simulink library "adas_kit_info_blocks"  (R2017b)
settings: Solver=ode1  StartTime=0.0  StopTime=Inf  FixedStep=0.001  RelTol=1e-3  EnableMultiTasking=on
PostLoadFcn:
  | , if any(exist('dsrtsu_mdlpostloadfcn', 'file') == [2, 3, 6]), try dsrtsu_mdlpostloadfcn('Execute', bdroot); catch fprintf('Error in PostLoadFcn (dsrtsu_mdlpostloadfcn) for model "%s":\n %s\n', bdroot, lasterr); end, end,
libraries: simulink x10, rtican x2

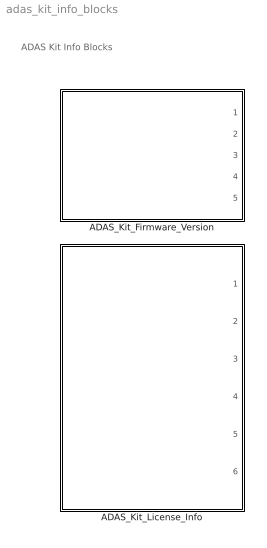
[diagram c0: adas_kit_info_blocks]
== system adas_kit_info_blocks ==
  note: ADAS Kit Info Blocks
  ADAS_Kit_Firmware_Version : Subsystem
  ADAS_Kit_License_Info : Subsystem

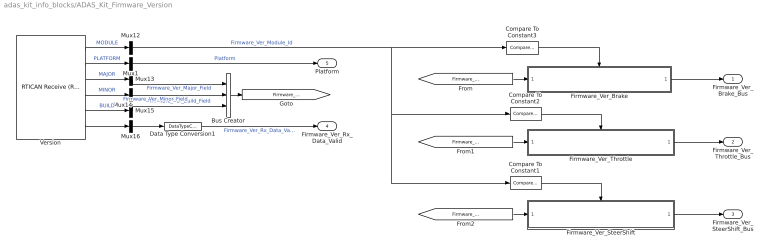
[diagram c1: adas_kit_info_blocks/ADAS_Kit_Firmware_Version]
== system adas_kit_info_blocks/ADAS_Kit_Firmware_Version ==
  Bus Creator : BusCreator  Inputs=3
  Compare To Constant1 : simulink/Logic and Bit Operations/Compare To Constant  relop===  const=3.0  OutDataTypeStr=boolean
  Compare To Constant2 : simulink/Logic and Bit Operations/Compare To Constant  relop===  const=2  OutDataTypeStr=boolean
  Compare To Constant3 : simulink/Logic and Bit Operations/Compare To Constant  relop===  const=1  OutDataTypeStr=boolean
  Data Type Conversion1 : DataTypeConversion  OutDataTypeStr=boolean
  Firmware_Ver_Brake : Subsystem  TreatAsAtomicUnit=on
  Firmware_Ver_SteerShift : Subsystem  TreatAsAtomicUnit=on
  Firmware_Ver_Throttle : Subsystem  TreatAsAtomicUnit=on
  Mux{1,12..16} (6 alike) : Mux  Inputs=1
  Version : rtican/RTICAN Receive (RX)   Reserved1=[]  Reserved2=[]  Reserved3=[]  Reserved4=[]  SfcnMessage=[]  Msg_Struct=[]  BoardTypeNo=[]  BoardNo=[]  ChannelNo=[]  Parameters=[]  DialogFcn=[]  UnitName=[]  Revision=[]  UnitValues=[]  DSProperties=struct('RTI',struct('Version',uint32(5),'BlockType',struct('isSLSource',uint8(1),'isSLSink',uint8(1),'isHWSource',uint8(0),'isHWSink',uint8(0),'isSetup',uint8(0),'isInline',uint8(1),'isNonInline',uint8(0),'isInterrupt',uint8(0),'isChannelwise',uint8(0)),'IOBoardType','RTICAN','UnitType','MESSAGE','Identifier','RX','DialogType','MSVC','BlockSet','RTICAN','SlaveProcessor','CAN'))  RTIBlockInterface=struct('OutputPortsWidth',int32([1 1 1 1 1 1]),'OutputPortsActive',[1 1 1 1 1 1],'OutputPortsName',{{'MODULE','PLATFORM','MAJOR','MINOR','BUILD',['RX status']}},'OutputPortsDataType',{{'SS_UINT8','SS_UINT8','SS_UINT16','SS_UINT16','SS_UINT16','SS_DOUBLE'}},'OutputPortsLabel',{{'MODULE','PLATFORM','MAJOR','MINOR','BUILD',''}},'OutputPortsLabelMode','ON','InputPortsWidth',int32(0),'InputPortsActive'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  RTIBlockParameters=struct('BoardTypeNo',{{1,'OFF',[]}},'BoardNo',{{1,'ON',[1 16]}},'ChannelNo',{{1,'ON',[1 2]}},'Parameters',{{struct('DataFileSupport',struct('DataFileSelectedMaster',1,'DataFileSelectedLocal',1,'DataFileName','c:\users\dataspeed\documents\matlab\dataspeed_dbw_dspace_simulink_library\lib\dataspeedbywire_19_oct_2017.dbc|','DataFileDate',['11-Jul-2018 12:27:42'],'SelectedFile','dataspeedbywire.dbc','I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  RTISFcnParameters=struct('SFcnRTICANMessage','struct','TLCFileName','char')  RTIBlockParaDefault=struct('BoardTypeNo',4302,'BoardNo',1,'ChannelNo',1,'Parameters',struct('DataFileSupport',struct('DataFileSelectedMaster',0,'DataFileSelectedLocal',0,'DataFileName','','DataFileDate','','SelectedFile',['<no file selected>']),'Options',struct('StatusSelected',1,'TimeSelected',1,'DeltaTimeSelected',1,'BytePortSelected',0,'MessageLengthSelected',0,'TriggerPort',struct('Selected',0,'TriggerType','risi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
  Firmware_Ver_Brake_Bus : Outport
  Firmware_Ver_Throttle_Bus : Outport  Port=2
  Firmware_Ver_SteerShift_Bus : Outport  Port=3
  Firmware_Ver_Rx_Data_Valid : Outport  Port=4
  Platform : Outport  Port=5
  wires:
  Data Type Conversion1/1 -> Firmware_Ver_Rx_Data_Valid/1  "Firmware_Ver_Rx_Data_Valid"
  Version/1 -> Mux12/1  "MODULE"
  Version/4 -> Mux14/1  "MINOR"
  Mux16/1 -> Data Type Conversion1/1
  Version/5 -> Mux15/1  "BUILD"
  Version/6 -> Mux16/1
  Mux12/1 -> Compare To Constant1/1, Compare To Constant2/1, Compare To Constant3/1  "Firmware_Ver_Module_Id"
  Version/3 -> Mux13/1  "MAJOR"
  Mux15/1 -> Bus Creator/3  "Firmware_Ver_Build_Field"
  Mux13/1 -> Bus Creator/1  "Firmware_Ver_Major_Field"
  Mux14/1 -> Bus Creator/2  "Firmware_Ver_Minor_Field"
  Compare To Constant1/1 -> Firmware_Ver_SteerShift/Enable
  Firmware_Ver_Brake/1(Firmware_Ver_Brake_Bus) -> Firmware_Ver_Brake_Bus/1
  Firmware_Ver_Throttle/1(Firmware_Ver_Throttle_Bus) -> Firmware_Ver_Throttle_Bus/1
  Firmware_Ver_SteerShift/1(Firmware_Ver_SteerShift_Bus) -> Firmware_Ver_SteerShift_Bus/1
  Compare To Constant2/1 -> Firmware_Ver_Throttle/Enable
  Compare To Constant3/1 -> Firmware_Ver_Brake/Enable
  Bus Creator/1 -> [Firmware_Ver_Info_Bus]
  [Firmware_Ver_Info_Bus] -> Firmware_Ver_Brake/1(Firmware_Ver_Info_Bus)
  [Firmware_Ver_Info_Bus] -> Firmware_Ver_Throttle/1(Firmware_Ver_Info_Bus)
  [Firmware_Ver_Info_Bus] -> Firmware_Ver_SteerShift/1(Firmware_Ver_Info_Bus)
  Version/2 -> Mux1/1  "PLATFORM"
  Mux1/1 -> Platform/1  "Platform"

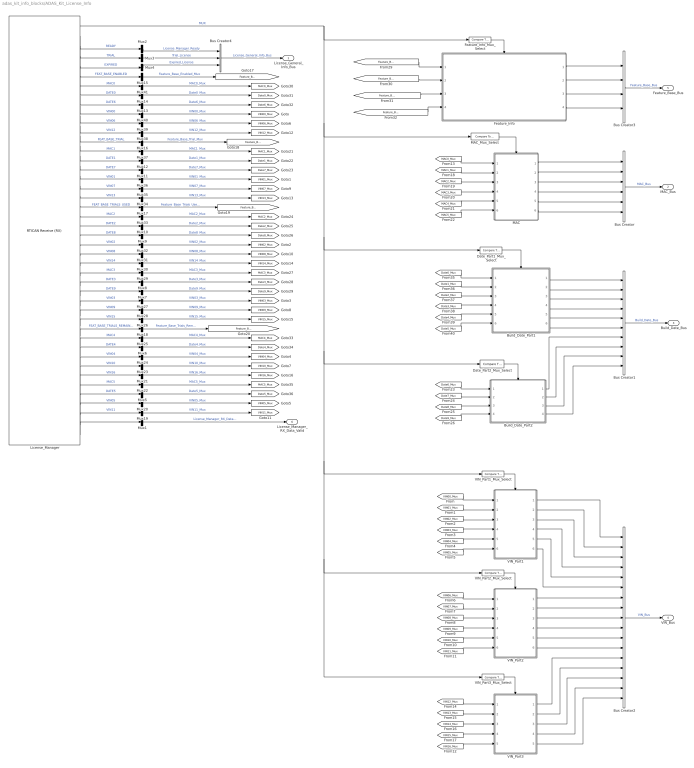
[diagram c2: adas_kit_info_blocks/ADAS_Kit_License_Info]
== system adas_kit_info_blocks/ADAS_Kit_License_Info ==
  Build_Date_Part1 : Subsystem
  Build_Date_Part2 : Subsystem
  Bus Creator : BusCreator  Inputs=6
  Bus Creator1 : BusCreator  Inputs=10
  Bus Creator2 : BusCreator  Inputs=17
  Bus Creator3 : BusCreator  Inputs=4
  Bus Creator4 : BusCreator  Inputs=3
  Date_Part1_Mux_Select : simulink/Logic and Bit Operations/Compare To Constant  relop===  const=129  OutDataTypeStr=boolean
  Date_Part2_Mux_Select : simulink/Logic and Bit Operations/Compare To Constant  relop===  const=130  OutDataTypeStr=boolean
  Feature_Info : Subsystem  AncestorBlock=dbw_interface_blocks/Subsystem/VIN_part1  TreatAsAtomicUnit=on
  Feature_Info_Mux_Select : simulink/Logic and Bit Operations/Compare To Constant  relop===  const=00  OutDataTypeStr=boolean
  License_Manager : rtican/RTICAN Receive (RX)   Reserved1=[]  Reserved2=[]  Reserved3=[]  Reserved4=[]  SfcnMessage=[]  Msg_Struct=[]  BoardTypeNo=[]  BoardNo=[]  ChannelNo=[]  Parameters=[]  DialogFcn=[]  UnitName=[]  Revision=[]  UnitValues=[]  DSProperties=struct('RTI',struct('Version',uint32(5),'BlockType',struct('isSLSource',uint8(1),'isSLSink',uint8(1),'isHWSource',uint8(0),'isHWSink',uint8(0),'isSetup',uint8(0),'isInline',uint8(1),'isNonInline',uint8(0),'isInterrupt',uint8(0),'isChannelwise',uint8(0)),'IOBoardType','RTICAN','UnitType','MESSAGE','Identifier','RX','DialogType','MSVC','BlockSet','RTICAN','SlaveProcessor','CAN'))  RTIBlockInterface=struct('OutputPortsWidth',int32([1 1 1 1 1 1 1 1 1 1 1 1 1 1 1 1 1 1 1 1 1 1 1 1 1 1 1 1 1 1 1 1 1 1 1 1 1 1 1 1 1 1]),'OutputPortsActive',ones(1,42),'OutputPortsName',{{'MUX','READY','TRIAL','EXPIRED','FEAT_BASE_ENABLED','MAC0','DATE0','DATE6','VIN00','VIN06','VIN12','FEAT_BASE_TRIAL','MAC1','DATE1','DATE7','VIN01','VIN07','VIN13','FEAT_BASE_TRIALS_USED','MAC2','DATE2','DATE8','VIN02','VIN08','VI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  RTIBlockParameters=struct('BoardTypeNo',{{1,'OFF',[]}},'BoardNo',{{1,'ON',[1 16]}},'ChannelNo',{{1,'ON',[1 2]}},'Parameters',{{struct('DataFileSupport',struct('DataFileSelectedMaster',1,'DataFileSelectedLocal',1,'DataFileName','c:\users\dataspeed\documents\matlab\dataspeed_dbw_dspace_simulink_library\lib\dataspeedbywire.dbc|','DataFileDate',['11-Jul-2018 12:27:42'],'SelectedFile','dataspeedbywire.dbc','InterfaceFcn'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  RTISFcnParameters=struct('SFcnRTICANMessage','struct','TLCFileName','char')  RTIBlockParaDefault=struct('BoardTypeNo',4302,'BoardNo',1,'ChannelNo',1,'Parameters',struct('DataFileSupport',struct('DataFileSelectedMaster',0,'DataFileSelectedLocal',0,'DataFileName','','DataFileDate','','SelectedFile',['<no file selected>']),'Options',struct('StatusSelected',1,'TimeSelected',1,'DeltaTimeSelected',1,'BytePortSelected',0,'MessageLengthSelected',0,'TriggerPort',struct('Selected',0,'TriggerType','risi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
  MAC : Subsystem
  MAC_Mux_Select : simulink/Logic and Bit Operations/Compare To Constant  relop===  const=128  OutDataTypeStr=boolean
  Mux{1..41} (41 alike) : Mux  Inputs=1
  VIN_Part1 : Subsystem  TreatAsAtomicUnit=on
  VIN_Part1_Mux_Select : simulink/Logic and Bit Operations/Compare To Constant  relop===  const=131  OutDataTypeStr=boolean
  VIN_Part2 : Subsystem  TreatAsAtomicUnit=on
  VIN_Part2_Mux_Select : simulink/Logic and Bit Operations/Compare To Constant  relop===  const=132  OutDataTypeStr=boolean
  VIN_Part3 : Subsystem  TreatAsAtomicUnit=on
  VIN_Part3_Mux_Select : simulink/Logic and Bit Operations/Compare To Constant  relop===  const=133  OutDataTypeStr=boolean
  License_General_Info_Bus : Outport
  MAC_Bus : Outport  Port=2
  Build_Date_Bus : Outport  Port=3
  VIN_Bus : Outport  Port=4
  Feature_Base_Bus : Outport  Port=5
  License_Manager_RX_Data_Valid : Outport  Port=6
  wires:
  License_Manager/23 -> Mux32/1  "VIN02"
  License_Manager/9 -> Mux40/1  "VIN00"
  [VIN04_Mux] -> VIN_Part1/5(VIN04_Mux)
  [VIN01_Mux] -> VIN_Part1/2(VIN01_Mux)
  [VIN13_Mux] -> VIN_Part3/2(VIN13_Mux)
  [VIN15_Mux] -> VIN_Part3/4(VIN15_Mux)
  [VIN12_Mux] -> VIN_Part3/1(VIN12_Mux)
  [VIN16_Mux] -> VIN_Part3/5(VIN16_Mux)
  VIN_Part3/4(VIN15) -> Bus Creator2/16
  [VIN14_Mux] -> VIN_Part3/3(VIN14_Mux)
  VIN_Part3_Mux_Select/1 -> VIN_Part3/Enable
  VIN_Part3/5(VIN16) -> Bus Creator2/17
  VIN_Part3/3(VIN14) -> Bus Creator2/15
  VIN_Part3/1(VIN12) -> Bus Creator2/13
  VIN_Part3/2(VIN13) -> Bus Creator2/14
  VIN_Part1_Mux_Select/1 -> VIN_Part1/Enable
  [VIN05_Mux] -> VIN_Part1/6(VIN05_Mux)
  [VIN03_Mux] -> VIN_Part1/4(VIN03_Mux)
  License_Manager/1 -> Feature_Info_Mux_Select/1, VIN_Part3_Mux_Select/1, VIN_Part2_Mux_Select/1, VIN_Part1_Mux_Select/1, Date_Part2_Mux_Select/1, Date_Part1_Mux_Select/1, MAC_Mux_Select/1  "MUX"
  VIN_Part1/3(VIN02) -> Bus Creator2/3
  VIN_Part1/6(VIN05) -> Bus Creator2/6
  [VIN00_Mux] -> VIN_Part1/1(VIN00_Mux)
  License_Manager/16 -> Mux36/1  "VIN01"
  License_Manager/3 -> Mux3/1  "TRIAL"
  License_Manager/4 -> Mux4/1  "EXPIRED"
  [VIN02_Mux] -> VIN_Part1/3(VIN02_Mux)
  License_Manager/5 -> Mux15/1  "FEAT_BASE_ENABLED"
  License_Manager/2 -> Mux2/1  "READY"
  License_Manager/13 -> Mux37/1  "MAC1"
  License_Manager/25 -> Mux30/1  "VIN14"
  License_Manager/30 -> Mux28/1  "VIN09"
  License_Manager/36 -> Mux23/1  "VIN10"
  License_Manager/12 -> Mux16/1  "FEAT_BASE_TRIAL"
  License_Manager/18 -> Mux34/1  "VIN13"
  License_Manager/32 -> Mux18/1  "FEAT_BASE_TRIALS_REMAINING"
  License_Manager/10 -> Mux39/1  "VIN06"
  License_Manager/24 -> Mux31/1  "VIN08"
  License_Manager/11 -> Mux38/1  "VIN12"
  License_Manager/31 -> Mux26/1  "VIN15"
  License_Manager/17 -> Mux35/1  "VIN07"
  License_Manager/19 -> Mux17/1  "FEAT_BASE_TRIALS_USED"
  License_Manager/41 -> Mux19/1  "VIN11"
  License_Manager/37 -> Mux21/1  "VIN16"
  License_Manager/42 -> Mux1/1
  VIN_Part2/6(VIN11) -> Bus Creator2/12
  VIN_Part2/5(VIN10) -> Bus Creator2/11
  [VIN10_Mux] -> VIN_Part2/5(VIN10_Mux)
  VIN_Part2/4(VIN09) -> Bus Creator2/10
  VIN_Part2/2(VIN07) -> Bus Creator2/8
  [VIN07_Mux] -> VIN_Part2/2(VIN07_Mux)
  VIN_Part2_Mux_Select/1 -> VIN_Part2/Enable
  [VIN08_Mux] -> VIN_Part2/3(VIN08_Mux)
  [VIN11_Mux] -> VIN_Part2/6(VIN11_Mux)
  VIN_Part2/1(VIN06) -> Bus Creator2/7
  VIN_Part2/3(VIN08) -> Bus Creator2/9
  [VIN06_Mux] -> VIN_Part2/1(VIN06_Mux)
  [VIN09_Mux] -> VIN_Part2/4(VIN09_Mux)
  License_Manager/29 -> Mux27/1  "VIN03"
  VIN_Part1/5(VIN04) -> Bus Creator2/5
  License_Manager/35 -> Mux24/1  "VIN04"
  VIN_Part1/1(VIN00) -> Bus Creator2/1
  VIN_Part1/2(VIN01) -> Bus Creator2/2
  VIN_Part1/4(VIN03) -> Bus Creator2/4
  License_Manager/40 -> Mux20/1  "VIN05"
  MAC/4(MAC3) -> Bus Creator/4
  MAC/2(MAC1) -> Bus Creator/2
  MAC/5(MAC4) -> Bus Creator/5
  [MAC2_Mux] -> MAC/3(MAC2_Mux)
  [MAC0_Mux] -> MAC/1(MAC0_Mux)
  MAC/6(MAC5) -> Bus Creator/6
  MAC/3(MAC2) -> Bus Creator/3
  [MAC3_Mux] -> MAC/4(MAC3_Mux)
  [MAC5_Mux] -> MAC/6(MAC5_Mux)
  [MAC1_Mux] -> MAC/2(MAC1_Mux)
  [MAC4_Mux] -> MAC/5(MAC4_Mux)
  [Date7_Mux] -> Build_Date_Part2/2(Date7_Mux)
  [Date9_Mux] -> Build_Date_Part2/4(Date9_Mux)
  Build_Date_Part2/3(Build_Date8) -> Bus Creator1/9
  [Date6_Mux] -> Build_Date_Part2/1(Date6_Mux)
  [Date8_Mux] -> Build_Date_Part2/3(Date8_Mux)
  Build_Date_Part2/1(Build_Date6) -> Bus Creator1/7
  Build_Date_Part2/2(Build_Date7) -> Bus Creator1/8
  Build_Date_Part2/4(Build_Date9) -> Bus Creator1/10
  Feature_Info/4(Feature_Base_Trials_Remaining) -> Bus Creator3/4
  Feature_Info/2(Feature_Base_Trial) -> Bus Creator3/2
  Feature_Info/1(Feature_Base_Enabled) -> Bus Creator3/1
  [Feature_Base_Trials_Used_Mux] -> Feature_Info/3(Feature_Base_Trials_Used_Mux)
  [Feature_Base_Enabled_Mux] -> Feature_Info/1(Feature_Base_Enabled_Mux)
  Feature_Info/3(Feature_Base_Trials_Used) -> Bus Creator3/3
  [Feature_Base_Trials_Remaining_Mux] -> Feature_Info/4(Feature_Base_Trials_Remaining_Mux)
  Feature_Info_Mux_Select/1 -> Feature_Info/Enable
  [Feature_Base_Trial_Mux] -> Feature_Info/2(Feature_Base_Trial_Mux)
  [Date4_Mux] -> Build_Date_Part1/5(Date4_Mux)
  [Date1_Mux] -> Build_Date_Part1/2(Date1_Mux)
  [Date5_Mux] -> Build_Date_Part1/6(Date5_Mux)
  [Date3_Mux] -> Build_Date_Part1/4(Date3_Mux)
  Build_Date_Part1/3(Build_Date2) -> Bus Creator1/3
  Build_Date_Part1/6(Build_Date5) -> Bus Creator1/6
  [Date0_Mux] -> Build_Date_Part1/1(Date0_Mux)
  [Date2_Mux] -> Build_Date_Part1/3(Date2_Mux)
  Build_Date_Part1/5(Build_Date4) -> Bus Creator1/5
  Build_Date_Part1/1(Build_Date0) -> Bus Creator1/1
  Build_Date_Part1/2(Build_Date1) -> Bus Creator1/2
  Build_Date_Part1/4(Build_Date3) -> Bus Creator1/4
  License_Manager/15 -> Mux11/1  "DATE7"
  License_Manager/14 -> Mux12/1  "DATE1"
  License_Manager/20 -> Mux33/1  "MAC2"
  License_Manager/21 -> Mux10/1  "DATE2"
  License_Manager/22 -> Mux9/1  "DATE8"
  License_Manager/26 -> Mux29/1  "MAC3"
  License_Manager/27 -> Mux8/1  "DATE3"
  License_Manager/28 -> Mux7/1  "DATE9"
  License_Manager/6 -> Mux41/1  "MAC0"
  License_Manager/7 -> Mux14/1  "DATE0"
  License_Manager/8 -> Mux13/1  "DATE6"
  License_Manager/33 -> Mux25/1  "MAC4"
  License_Manager/34 -> Mux6/1  "DATE4"
  License_Manager/38 -> Mux22/1  "MAC5"
  License_Manager/39 -> Mux5/1  "DATE5"
  Date_Part1_Mux_Select/1 -> Build_Date_Part1/Enable
  Date_Part2_Mux_Select/1 -> Build_Date_Part2/Enable
  MAC_Mux_Select/1 -> MAC/Enable
  Mux1/1 -> License_Manager_RX_Data_Valid/1  "License_Manager_RX_Data_Valid"
  Mux2/1 -> Bus Creator4/1  "License_Manager_Ready"
  Mux3/1 -> Bus Creator4/2  "Trial_License"
  Mux4/1 -> Bus Creator4/3  "Expired_License"
  Mux5/1 -> [Date5_Mux]  "Date5_Mux"
  Mux6/1 -> [Date4_Mux]  "Date4_Mux"
  Mux7/1 -> [Date9_Mux]  "Date9_Mux"
  Mux8/1 -> [Date3_Mux]  "Date3_Mux"
  Mux9/1 -> [Date8_Mux]  "Date8_Mux"
  Mux10/1 -> [Date2_Mux]  "Date2_Mux"
  Mux11/1 -> [Date7_Mux]  "Date7_Mux"
  Mux12/1 -> [Date1_Mux]  "Date1_Mux"
  Mux13/1 -> [Date6_Mux]  "Date6_Mux"
  Mux14/1 -> [Date0_Mux]  "Date0_Mux"
  Mux15/1 -> [Feature_Base_Enabled_Mux]  "Feature_Base_Enabled_Mux"
  Mux16/1 -> [Feature_Base_Trial_Mux]  "Feature_Base_Trial_Mux"
  Mux17/1 -> [Feature_Base_Trials_Used_Mux]  "Feature_Base_Trials_Used_Mux"
  Mux18/1 -> [Feature_Base_Trials_Remaining_Mux]  "Feature_Base_Trials_Remaining_Mux"
  Bus Creator/1 -> MAC_Bus/1  "MAC_Bus"
  MAC/1(MAC0) -> Bus Creator/1
  Bus Creator1/1 -> Build_Date_Bus/1  "Build_Date_Bus"
  Bus Creator2/1 -> VIN_Bus/1  "VIN_Bus"
  Bus Creator3/1 -> Feature_Base_Bus/1  "Feature_Base_Bus"
  Bus Creator4/1 -> License_General_Info_Bus/1  "License_General_Info_Bus"
  Mux19/1 -> [VIN11_Mux]  "VIN11_Mux"
  Mux20/1 -> [VIN05_Mux]  "VIN05_Mux"
  Mux21/1 -> [VIN16_Mux]  "VIN16_Mux"
  Mux22/1 -> [MAC5_Mux]  "MAC5_Mux"
  Mux23/1 -> [VIN10_Mux]  "VIN10_Mux"
  Mux24/1 -> [VIN04_Mux]  "VIN04_Mux"
  Mux25/1 -> [MAC4_Mux]  "MAC4_Mux"
  Mux26/1 -> [VIN15_Mux]  "VIN15_Mux"
  Mux27/1 -> [VIN03_Mux]  "VIN03_Mux"
  Mux28/1 -> [VIN09_Mux]  "VIN09_Mux"
  Mux29/1 -> [MAC3_Mux]  "MAC3_Mux"
  Mux30/1 -> [VIN14_Mux]  "VIN14_Mux"
  Mux31/1 -> [VIN08_Mux]  "VIN08_Mux"
  Mux32/1 -> [VIN02_Mux]  "VIN02_Mux"
  Mux33/1 -> [MAC2_Mux]  "MAC2_Mux"
  Mux34/1 -> [VIN13_Mux]  "VIN13_Mux"
  Mux35/1 -> [VIN07_Mux]  "VIN07_Mux"
  Mux36/1 -> [VIN01_Mux]  "VIN01_Mux"
  Mux37/1 -> [MAC1_Mux]  "MAC1_Mux"
  Mux38/1 -> [VIN12_Mux]  "VIN12_Mux"
  Mux39/1 -> [VIN06_Mux]  "VIN06_Mux"
  Mux40/1 -> [VIN00_Mux]  "VIN00_Mux"
  Mux41/1 -> [MAC0_Mux]  "MAC0_Mux"

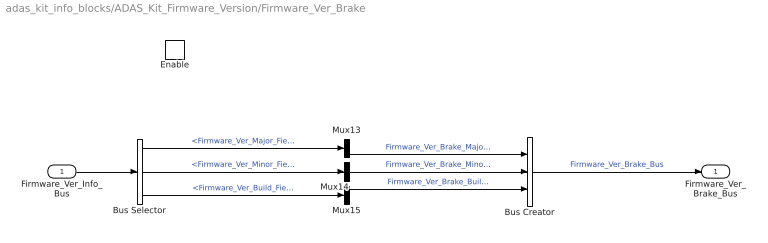
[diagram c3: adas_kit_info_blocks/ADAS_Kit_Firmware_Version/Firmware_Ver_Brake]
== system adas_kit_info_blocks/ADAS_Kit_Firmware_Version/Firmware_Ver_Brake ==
  Firmware_Ver_Info_Bus : Inport
  Enable : EnablePort
  Bus Creator : BusCreator  Inputs=3
  Bus Selector : BusSelector  OutputSignals=Firmware_Ver_Major_Field,Firmware_Ver_Minor_Field,Firmware_Ver_Build_Field
  Mux13 : Mux  Inputs=1
  Mux14 : Mux  Inputs=1
  Mux15 : Mux  Inputs=1
  Firmware_Ver_Brake_Bus : Outport
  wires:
  Firmware_Ver_Info_Bus/1 -> Bus Selector/1
  Mux14/1 -> Bus Creator/2  "Firmware_Ver_Brake_Minor_Field"
  Mux13/1 -> Bus Creator/1  "Firmware_Ver_Brake_Major_Field"
  Mux15/1 -> Bus Creator/3  "Firmware_Ver_Brake_Build_Field"
  Bus Selector/1 -> Mux13/1  "<Firmware_Ver_Major_Field>"
  Bus Selector/2 -> Mux14/1  "<Firmware_Ver_Minor_Field>"
  Bus Selector/3 -> Mux15/1  "<Firmware_Ver_Build_Field>"
  Bus Creator/1 -> Firmware_Ver_Brake_Bus/1  "Firmware_Ver_Brake_Bus"

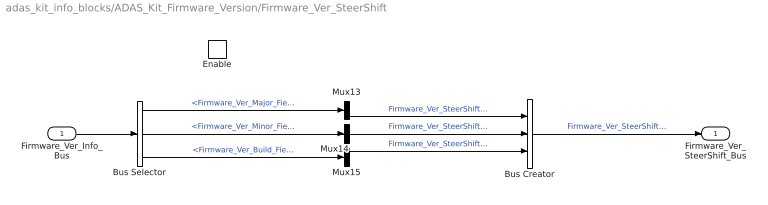
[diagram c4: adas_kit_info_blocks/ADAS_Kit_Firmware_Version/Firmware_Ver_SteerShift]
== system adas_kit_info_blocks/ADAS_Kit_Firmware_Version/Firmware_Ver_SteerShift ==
  Firmware_Ver_Info_Bus : Inport
  Enable : EnablePort
  Bus Creator : BusCreator  Inputs=3
  Bus Selector : BusSelector  OutputSignals=Firmware_Ver_Major_Field,Firmware_Ver_Minor_Field,Firmware_Ver_Build_Field
  Mux13 : Mux  Inputs=1
  Mux14 : Mux  Inputs=1
  Mux15 : Mux  Inputs=1
  Firmware_Ver_SteerShift_Bus : Outport
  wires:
  Mux15/1 -> Bus Creator/3  "Firmware_Ver_SteerShift_Build_Field"
  Bus Selector/3 -> Mux15/1  "<Firmware_Ver_Build_Field>"
  Mux13/1 -> Bus Creator/1  "Firmware_Ver_SteerShift_Major_Field"
  Bus Creator/1 -> Firmware_Ver_SteerShift_Bus/1  "Firmware_Ver_SteerShift_Bus"
  Bus Selector/2 -> Mux14/1  "<Firmware_Ver_Minor_Field>"
  Bus Selector/1 -> Mux13/1  "<Firmware_Ver_Major_Field>"
  Mux14/1 -> Bus Creator/2  "Firmware_Ver_SteerShift_Minor_Field"
  Firmware_Ver_Info_Bus/1 -> Bus Selector/1

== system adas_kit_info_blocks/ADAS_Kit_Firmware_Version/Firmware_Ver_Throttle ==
  Firmware_Ver_Info_Bus : Inport
  Enable : EnablePort
  Bus Creator : BusCreator  Inputs=3
  Bus Selector : BusSelector  OutputSignals=Firmware_Ver_Major_Field,Firmware_Ver_Minor_Field,Firmware_Ver_Build_Field
  Mux13 : Mux  Inputs=1
  Mux14 : Mux  Inputs=1
  Mux15 : Mux  Inputs=1
  Firmware_Ver_Throttle_Bus : Outport
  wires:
  Mux15/1 -> Bus Creator/3  "Firmware_Ver_Throttle_Build_Field"
  Bus Selector/3 -> Mux15/1  "<Firmware_Ver_Build_Field>"
  Mux13/1 -> Bus Creator/1  "Firmware_Ver_Throttle_Major_Field"
  Bus Creator/1 -> Firmware_Ver_Throttle_Bus/1  "Firmware_Ver_Throttle_Bus"
  Bus Selector/2 -> Mux14/1  "<Firmware_Ver_Minor_Field>"
  Bus Selector/1 -> Mux13/1  "<Firmware_Ver_Major_Field>"
  Mux14/1 -> Bus Creator/2  "Firmware_Ver_Throttle_Minor_Field"
  Firmware_Ver_Info_Bus/1 -> Bus Selector/1

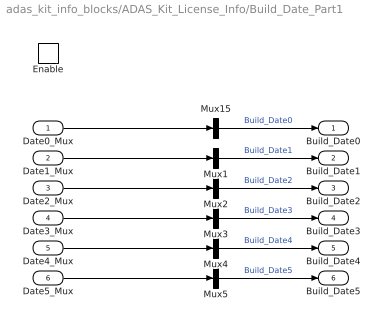
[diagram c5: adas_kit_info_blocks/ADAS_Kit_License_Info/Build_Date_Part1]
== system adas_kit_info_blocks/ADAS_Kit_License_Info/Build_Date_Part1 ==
  Date0_Mux : Inport
  Date1_Mux : Inport  Port=2
  Date2_Mux : Inport  Port=3
  Date3_Mux : Inport  Port=4
  Date4_Mux : Inport  Port=5
  Date5_Mux : Inport  Port=6
  Enable : EnablePort
  Mux{1..5,15} (6 alike) : Mux  Inputs=1
  Build_Date0 : Outport
  Build_Date1 : Outport  Port=2
  Build_Date2 : Outport  Port=3
  Build_Date3 : Outport  Port=4
  Build_Date4 : Outport  Port=5
  Build_Date5 : Outport  Port=6
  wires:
  Date0_Mux/1 -> Mux15/1
  Date1_Mux/1 -> Mux1/1
  Date3_Mux/1 -> Mux3/1
  Date4_Mux/1 -> Mux4/1
  Date5_Mux/1 -> Mux5/1
  Date2_Mux/1 -> Mux2/1
  Mux15/1 -> Build_Date0/1  "Build_Date0"
  Mux1/1 -> Build_Date1/1  "Build_Date1"
  Mux2/1 -> Build_Date2/1  "Build_Date2"
  Mux3/1 -> Build_Date3/1  "Build_Date3"
  Mux4/1 -> Build_Date4/1  "Build_Date4"
  Mux5/1 -> Build_Date5/1  "Build_Date5"

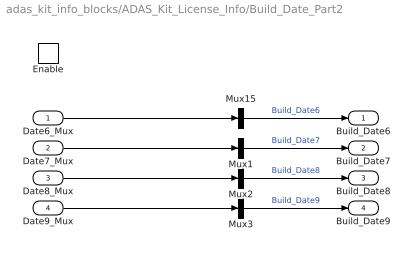
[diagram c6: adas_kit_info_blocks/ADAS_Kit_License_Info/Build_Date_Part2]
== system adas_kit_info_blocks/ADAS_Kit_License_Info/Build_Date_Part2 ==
  Date6_Mux : Inport
  Date7_Mux : Inport  Port=2
  Date8_Mux : Inport  Port=3
  Date9_Mux : Inport  Port=4
  Enable : EnablePort
  Mux{1..3,15} (4 alike) : Mux  Inputs=1
  Build_Date6 : Outport
  Build_Date7 : Outport  Port=2
  Build_Date8 : Outport  Port=3
  Build_Date9 : Outport  Port=4
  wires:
  Date8_Mux/1 -> Mux2/1
  Date9_Mux/1 -> Mux3/1
  Date6_Mux/1 -> Mux15/1
  Date7_Mux/1 -> Mux1/1
  Mux15/1 -> Build_Date6/1  "Build_Date6"
  Mux1/1 -> Build_Date7/1  "Build_Date7"
  Mux2/1 -> Build_Date8/1  "Build_Date8"
  Mux3/1 -> Build_Date9/1  "Build_Date9"

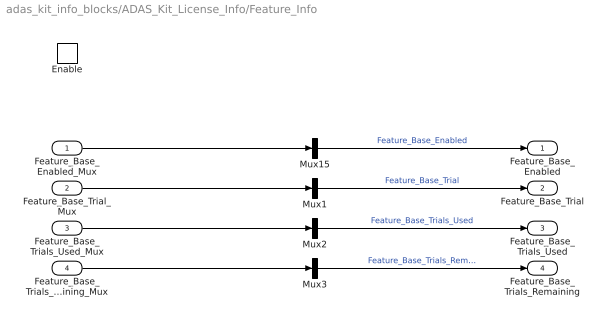
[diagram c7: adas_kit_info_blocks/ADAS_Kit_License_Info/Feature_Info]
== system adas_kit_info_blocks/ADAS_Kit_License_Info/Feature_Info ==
  Feature_Base_Enabled_Mux : Inport
  Feature_Base_Trial_Mux : Inport  Port=2
  Feature_Base_Trials_Used_Mux : Inport  Port=3
  Feature_Base_Trials_Remaining_Mux : Inport  Port=4
  Enable : EnablePort
  Mux{1..3,15} (4 alike) : Mux  Inputs=1
  Feature_Base_Enabled : Outport
  Feature_Base_Trial : Outport  Port=2
  Feature_Base_Trials_Used : Outport  Port=3
  Feature_Base_Trials_Remaining : Outport  Port=4
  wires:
  Mux3/1 -> Feature_Base_Trials_Remaining/1  "Feature_Base_Trials_Remaining"
  Mux2/1 -> Feature_Base_Trials_Used/1  "Feature_Base_Trials_Used"
  Mux1/1 -> Feature_Base_Trial/1  "Feature_Base_Trial"
  Mux15/1 -> Feature_Base_Enabled/1  "Feature_Base_Enabled"
  Feature_Base_Enabled_Mux/1 -> Mux15/1
  Feature_Base_Trials_Remaining_Mux/1 -> Mux3/1
  Feature_Base_Trials_Used_Mux/1 -> Mux2/1
  Feature_Base_Trial_Mux/1 -> Mux1/1

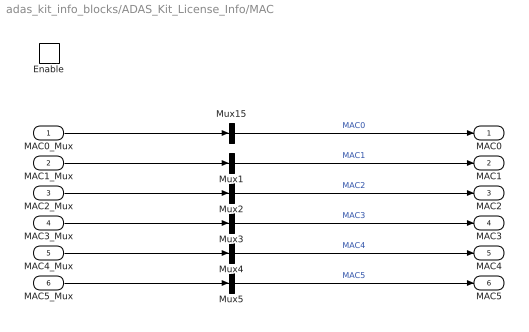
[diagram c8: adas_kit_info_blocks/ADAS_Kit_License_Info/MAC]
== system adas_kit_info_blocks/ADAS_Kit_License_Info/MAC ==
  MAC0_Mux : Inport
  MAC1_Mux : Inport  Port=2
  MAC2_Mux : Inport  Port=3
  MAC3_Mux : Inport  Port=4
  MAC4_Mux : Inport  Port=5
  MAC5_Mux : Inport  Port=6
  Enable : EnablePort
  Mux{1..5,15} (6 alike) : Mux  Inputs=1
  MAC0 : Outport
  MAC1 : Outport  Port=2
  MAC2 : Outport  Port=3
  MAC3 : Outport  Port=4
  MAC4 : Outport  Port=5
  MAC5 : Outport  Port=6
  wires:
  MAC0_Mux/1 -> Mux15/1
  MAC1_Mux/1 -> Mux1/1
  MAC4_Mux/1 -> Mux4/1
  MAC2_Mux/1 -> Mux2/1
  MAC3_Mux/1 -> Mux3/1
  MAC5_Mux/1 -> Mux5/1
  Mux15/1 -> MAC0/1  "MAC0"
  Mux1/1 -> MAC1/1  "MAC1"
  Mux2/1 -> MAC2/1  "MAC2"
  Mux3/1 -> MAC3/1  "MAC3"
  Mux4/1 -> MAC4/1  "MAC4"
  Mux5/1 -> MAC5/1  "MAC5"

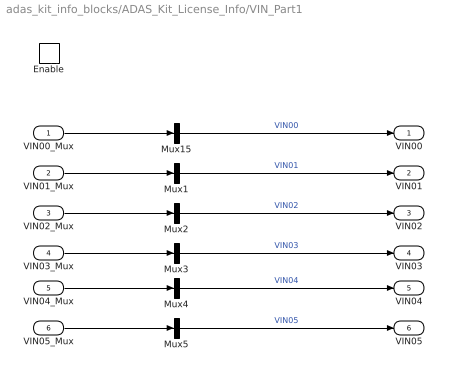
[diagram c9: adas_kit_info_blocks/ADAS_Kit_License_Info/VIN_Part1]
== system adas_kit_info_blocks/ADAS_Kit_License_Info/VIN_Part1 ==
  VIN00_Mux : Inport
  VIN01_Mux : Inport  Port=2
  VIN02_Mux : Inport  Port=3
  VIN03_Mux : Inport  Port=4
  VIN04_Mux : Inport  Port=5
  VIN05_Mux : Inport  Port=6
  Enable : EnablePort
  Mux{1..5,15} (6 alike) : Mux  Inputs=1
  VIN00 : Outport
  VIN01 : Outport  Port=2
  VIN02 : Outport  Port=3
  VIN03 : Outport  Port=4
  VIN04 : Outport  Port=5
  VIN05 : Outport  Port=6
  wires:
  Mux15/1 -> VIN00/1  "VIN00"
  Mux1/1 -> VIN01/1  "VIN01"
  Mux2/1 -> VIN02/1  "VIN02"
  Mux3/1 -> VIN03/1  "VIN03"
  Mux4/1 -> VIN04/1  "VIN04"
  Mux5/1 -> VIN05/1  "VIN05"
  VIN00_Mux/1 -> Mux15/1
  VIN01_Mux/1 -> Mux1/1
  VIN02_Mux/1 -> Mux2/1
  VIN03_Mux/1 -> Mux3/1
  VIN04_Mux/1 -> Mux4/1
  VIN05_Mux/1 -> Mux5/1

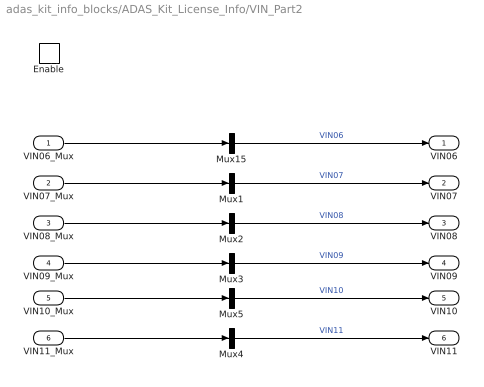
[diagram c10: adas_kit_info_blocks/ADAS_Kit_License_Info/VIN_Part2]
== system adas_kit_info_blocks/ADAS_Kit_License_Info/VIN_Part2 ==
  VIN06_Mux : Inport
  VIN07_Mux : Inport  Port=2
  VIN08_Mux : Inport  Port=3
  VIN09_Mux : Inport  Port=4
  VIN10_Mux : Inport  Port=5
  VIN11_Mux : Inport  Port=6
  Enable : EnablePort
  Mux{1..5,15} (6 alike) : Mux  Inputs=1
  VIN06 : Outport
  VIN07 : Outport  Port=2
  VIN08 : Outport  Port=3
  VIN09 : Outport  Port=4
  VIN10 : Outport  Port=5
  VIN11 : Outport  Port=6
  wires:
  Mux4/1 -> VIN11/1  "VIN11"
  Mux5/1 -> VIN10/1  "VIN10"
  Mux3/1 -> VIN09/1  "VIN09"
  Mux2/1 -> VIN08/1  "VIN08"
  Mux1/1 -> VIN07/1  "VIN07"
  Mux15/1 -> VIN06/1  "VIN06"
  VIN11_Mux/1 -> Mux4/1
  VIN10_Mux/1 -> Mux5/1
  VIN06_Mux/1 -> Mux15/1
  VIN07_Mux/1 -> Mux1/1
  VIN08_Mux/1 -> Mux2/1
  VIN09_Mux/1 -> Mux3/1

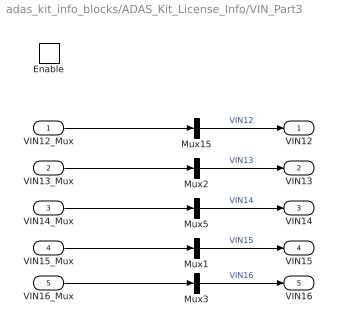
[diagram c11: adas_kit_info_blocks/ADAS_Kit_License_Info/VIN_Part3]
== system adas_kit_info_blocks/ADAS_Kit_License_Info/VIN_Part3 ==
  VIN12_Mux : Inport
  VIN13_Mux : Inport  Port=2
  VIN14_Mux : Inport  Port=3
  VIN15_Mux : Inport  Port=4
  VIN16_Mux : Inport  Port=5
  Enable : EnablePort
  Mux{1..3,5,15} (5 alike) : Mux  Inputs=1
  VIN12 : Outport
  VIN13 : Outport  Port=2
  VIN14 : Outport  Port=3
  VIN15 : Outport  Port=4
  VIN16 : Outport  Port=5
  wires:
  Mux15/1 -> VIN12/1  "VIN12"
  Mux2/1 -> VIN13/1  "VIN13"
  Mux5/1 -> VIN14/1  "VIN14"
  Mux1/1 -> VIN15/1  "VIN15"
  Mux3/1 -> VIN16/1  "VIN16"
  VIN16_Mux/1 -> Mux3/1
  VIN15_Mux/1 -> Mux1/1
  VIN14_Mux/1 -> Mux5/1
  VIN13_Mux/1 -> Mux2/1
  VIN12_Mux/1 -> Mux15/1
